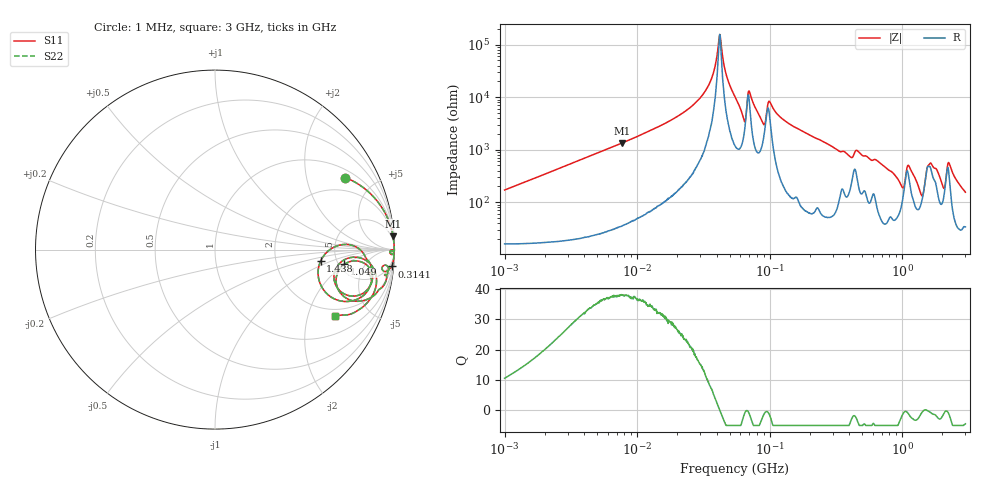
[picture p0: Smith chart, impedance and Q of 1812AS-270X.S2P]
!s-Parameter Generated by FASTRON Sdn. Bhd.
!FASTRON P/N : 1812AS-270X
!Keysight Technologies,E4991B,MY54100416,A.01.15
!Date created: Mon Oct 16 10:00:43 2023
!Version  : Rev00 Mon Oct 16 10:00:43 2023
!Data & Calibration Information:
!Freq	S11	S21	S12	S22
!PortZ  Port1:50+j0  Port2:50+j0
!When reading, reference impedance value at option line is always used.
! Remarks : This data is being provided solely for informational purposes.
# Hz S dB R 50
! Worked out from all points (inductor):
!   1601 points, 1 MHz to 3 GHz, reference 50 ohm
!   read as one part in series: L = 26.9 uH near 1.041 MHz
!   highest Q = 37.9 at 7.665 MHz (marker M1), where L = 27.7 uH
!   self-resonance near 42.01 MHz
!   S11 on the Smith chart (normalised r, x): 1 MHz: 1.32, +3.39; 314.1 MHz: 2, -21; 1.049 GHz: 5.57, -1.93; 1.438 GHz: 3.74, -0.74; 3 GHz: 1.68, -3.02
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1000000  -1.63 29.0  -6.26 -55.6  -6.26 -55.6  -1.63 29.0
3804036  -0.14 8.7  -16.37 -79.4  -16.37 -79.4  -0.14 8.7
7664657  -0.04 4.3  -22.54 -84.2  -22.54 -84.2  -0.04 4.3
1.447069e7  -0.02 2.1  -28.74 -86.1  -28.74 -86.1  -0.02 2.1
3.142935e7  -0.01 0.5  -41.09 -85.2  -41.09 -85.2  -0.01 0.5
3.707242e7  -0.01 0.2  -48.15 -80.7  -48.15 -80.7  -0.01 0.2
4.201274e7  -0.01 0.0  -63.87 -1.7  -63.87 -1.7  -0.01 0.0
5.477226e7  -0.01 -0.6  -40.14 82.7  -40.14 82.7  -0.01 -0.6
6.364388e7  -0.11 -1.3  -31.79 61.5  -31.79 61.5  -0.11 -1.3
7.105049e7  -0.04 -0.4  -41.49 60.3  -41.49 60.3  -0.04 -0.4
8.899408e7  -0.12 -1.6  -30.16 61.9  -30.16 61.9  -0.12 -1.6
1.008535e8  -0.05 -0.6  -38.05 63.3  -38.05 63.3  -0.05 -0.6
2.083556e8  -0.03 -3.2  -25.15 84.9  -25.15 84.9  -0.03 -3.2
3.140564e8  -0.09 -5.4  -20.46 81.1  -20.46 81.1  -0.09 -5.4
7.925923e8  -0.48 -13.3  -12.68 70.0  -12.68 70.0  -0.48 -13.3
1.048936e9  -2.80 -6.5  -10.69 16.4  -10.69 16.4  -2.80 -6.5
1.125055e9  -1.07 -8.5  -14.83 46.3  -14.83 46.3  -1.07 -8.5
1.437675e9  -4.56 -6.3  -7.60 8.9  -7.60 8.9  -4.56 -6.3
1.596974e9  -1.44 -3.6  -15.75 19.2  -15.75 19.2  -1.44 -3.6
2.03054e9  -2.52 -18.7  -8.46 39.5  -8.46 39.5  -2.52 -18.7
2.255531e9  -0.96 -7.4  -15.91 45.8  -15.91 45.8  -0.96 -7.4
3e9  -2.31 -28.9  -6.10 48.4  -6.10 48.4  -2.31 -28.9
